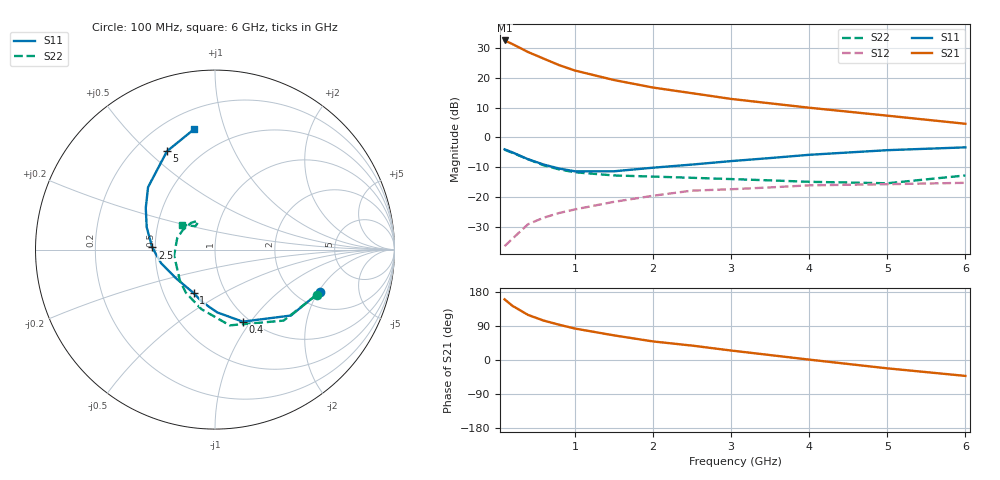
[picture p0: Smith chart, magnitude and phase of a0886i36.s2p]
!  MSA-0886 S AND NOISE PARAMETERS
!  Id=36mA  LAST UPDATED 07-27-92
# ghz s ma r 50
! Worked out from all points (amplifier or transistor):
!   14 points, 100 MHz to 6 GHz, reference 50 ohm
!   highest |S21| = 32.5 dB at 100 MHz (marker M1)
!   |S21| within 3 dB of that: start of sweep to 334.2 MHz
!   unconditionally stable (mu >= 1): 2.836 GHz to 5.63 GHz
!   at 400 MHz: K = 0.68, MSG = 28.9 dB, |S12| = -29.1 dB
!   at 2 GHz: K = 0.96, MSG = 18.1 dB, |S12| = -19.6 dB
!   at 6 GHz: K = 0.99, MSG = 9.9 dB, |S12| = -15.2 dB
!   lowest NFmin = 2.70 dB at 100 MHz
!   S11 on the Smith chart (normalised r, x): 100 MHz: 2.64, -2.06; 400 MHz: 0.93, -0.92; 1 GHz: 0.71, -0.37; 2.5 GHz: 0.48, +0.01; 5 GHz: 0.33, +0.58; 6 GHz: 0.32, +0.79
0.1  0.63 -22.0  42.12 160.0  0.015 54.0  0.62 -24.0
0.2  0.56 -41.0  36.68 143.0  0.02 50.0  0.55 -46.0
0.4  0.43 -69.0  26.94 119.0  0.035 52.0  0.43 -79.0
0.6  0.35 -88.0  20.89 104.0  0.045 49.0  0.34 -103.0
0.8  0.3 -104.0  16.21 93.0  0.054 50.0  0.29 -124.0
1  0.27 -116.0  13.2 83.0  0.062 49.0  0.26 -139.0
1.5  0.27 -144.0  9.15 65.0  0.083 46.0  0.23 -172.0
2  0.31 -166.0  6.84 49.0  0.105 41.0  0.22 163.0
2.5  0.35 178.0  5.5 38.0  0.128 36.0  0.21 149.0
3  0.4 162.0  4.41 25.0  0.135 30.0  0.2 132.0
3.5  0.45 149.0  3.72 13.0  0.145 25.0  0.19 124.0
4  0.51 137.0  3.14 1.0  0.157 19.0  0.18 121.0
5  0.61 116.0  2.31 -22.0  0.164 10.0  0.17 130.0
6  0.68 100.0  1.69 -42.0  0.173 4.0  0.23 143.0
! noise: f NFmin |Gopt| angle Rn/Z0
0.1  2.7  0.36  1  0.63
0.5  2.9  0.35  4  0.63
1  3.1  0.32  7  0.63
2  3.6  0.22  6  0.61
